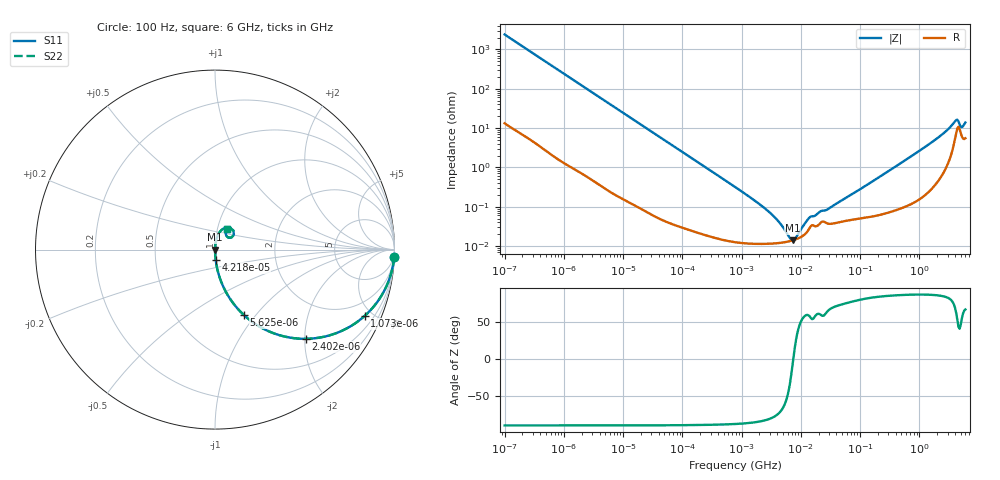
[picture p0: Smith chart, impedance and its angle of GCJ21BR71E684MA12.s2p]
!Murata Part Number: GCJ21BR71E684MA12
!These Parameters are Measured in Series Mode Connection
!Data Generated on Mar 13, 2026
!  o--ll--o
!Port1  Port2
!  o------o
!Operation Temp=25[degC], DC Bias Voltage=0[V]
!Freq. Start=100[Hz] Stop=6[GHz] 401[Steps]
# Hz S RI R 50
!Freq.(Hz) S11(Real) S11(Imag) S21(Real) S21(Imag) S12(Real) S12(Imag) S22(Real) S22(Imag)
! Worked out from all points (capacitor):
!   401 points, 100 Hz to 6 GHz, reference 50 ohm
!   read as one part in series: C = 660 nF near 109 Hz
!   lowest |Z| = 14 mohm at 7.267 MHz (marker M1)
!   series resonance near 7.466 MHz, so ESL is about 690 pH
!   S11 on the Smith chart (normalised r, x): 100 Hz: 1, -48; 1.073 kHz: 1.02, -4.52; 2.402 kHz: 1.01, -2.03; 5.625 kHz: 1.01, -0.87; 42.18 kHz: 1.00, -0.12; 6 GHz: 1.11, +0.25
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100  0.998 -0.0415  0.00195 0.0415  0.00195 0.0415  0.998 -0.0415
350  0.9787 -0.1417  0.0213 0.1417  0.0213 0.1417  0.9787 -0.1417
1073  0.8351 -0.3684  0.1649 0.3684  0.1649 0.3684  0.8351 -0.3684
2008  0.5939 -0.4882  0.4061 0.4882  0.4061 0.4882  0.5939 -0.4882
2402  0.5064 -0.4971  0.4936 0.4971  0.4936 0.4971  0.5064 -0.4971
5625  0.1599 -0.3636  0.8401 0.3636  0.8401 0.3636  0.1599 -0.3636
12041  0.0408 -0.1947  0.9592 0.1947  0.9592 0.1947  0.0408 -0.1947
40335  0.0042 -0.0607  0.9958 0.0607  0.9958 0.0607  0.0042 -0.0607
42182  0.00387 -0.058  0.9961 0.058  0.9961 0.058  0.00387 -0.058
774597  0.000135 -0.00319  0.9999 0.00319  0.9999 0.00319  0.000135 -0.00319
3103719  0.000115 -0.000666  0.9999 0.000666  0.9999 0.000666  0.000115 -0.000666
6644369  0.000134 -7.81e-05  0.9999 7.81e-05  0.9999 7.81e-05  0.000134 -7.81e-05
7266822  0.000139 -1.8e-05  0.9999 1.8e-05  0.9999 1.8e-05  0.000139 -1.8e-05
8311524  0.000149 7.23e-05  0.9999 -7.23e-05  0.9999 -7.23e-05  0.000149 7.23e-05
1.300572e7  0.000238 0.0004  0.9998 -0.0004  0.9998 -0.0004  0.000238 0.0004
1.555665e7  0.00034 0.000459  0.9997 -0.000459  0.9997 -0.000459  0.00034 0.000459
2.911731e7  0.00037 0.000798  0.9996 -0.000798  0.9996 -0.000798  0.00037 0.000798
3.124326e8  0.000788 0.00828  0.9992 -0.00828  0.9992 -0.00828  0.000788 0.00828
1.873145e9  0.00619 0.0504  0.9938 -0.0504  0.9938 -0.0504  0.00619 0.0504
4.009986e9  0.0674 0.1234  0.9326 -0.1234  0.9326 -0.1234  0.0674 0.1234
5.245841e9  0.0632 0.0762  0.9368 -0.0762  0.9368 -0.0762  0.0632 0.0762
6e9  0.0658 0.1125  0.9342 -0.1125  0.9342 -0.1125  0.0658 0.1125
